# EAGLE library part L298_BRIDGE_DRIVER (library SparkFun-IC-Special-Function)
Full-bridge power driver IC
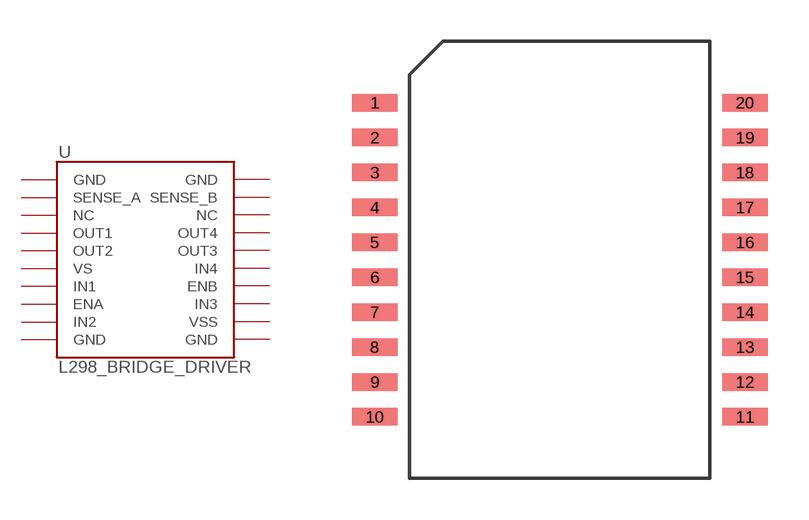
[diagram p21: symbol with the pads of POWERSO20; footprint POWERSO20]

Designator prefix -

## L298_BRIDGE_DRIVER (PROD_ID: IC-09133; VALUE: L298P013)  [POWERSO20]
1  GND
2  SENSE_A
3  NC
4  OUT1
5  OUT2
6  VS
7  IN1
8  ENA
9  IN2
10  GND
11  GND
12  VSS
13  IN3
14  ENB
15  IN4
16  OUT3
17  OUT4
18  NC
19  SENSE_B
20  GND

## Footprint POWERSO20 (pad centres in mm)
smd 1.651 x 0.635: 1 -6.731,5.715; 2 -6.731,4.445; 3 -6.731,3.175; 4 -6.731,1.905; 5 -6.731,0.635; 6 -6.731,-0.635; 7 -6.731,-1.905; 8 -6.731,-3.175; 9 -6.731,-4.445; 10 -6.731,-5.715; 11 6.731,-5.715; 12 6.731,-4.445; 13 6.731,-3.175; 14 6.731,-1.905; 15 6.731,-0.635; 16 6.731,0.635; 17 6.731,1.905; 18 6.731,3.175; 19 6.731,4.445; 20 6.731,5.715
